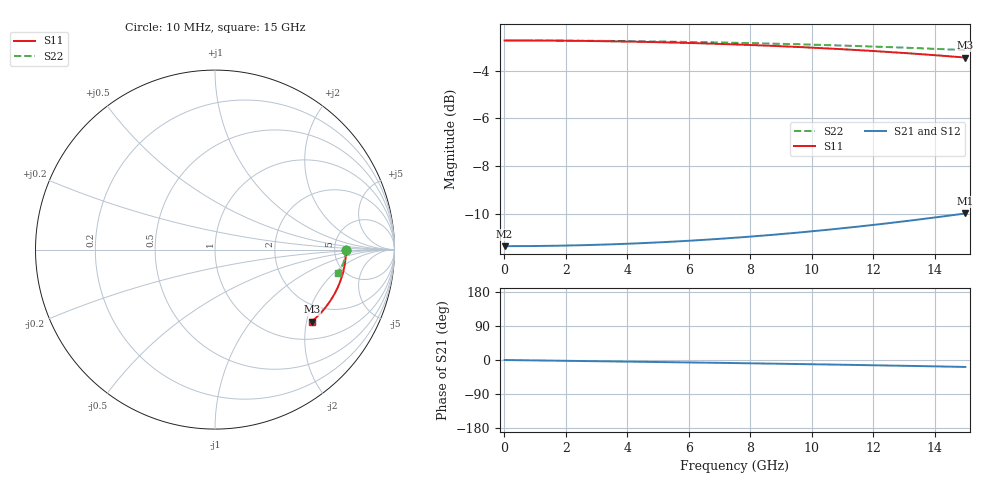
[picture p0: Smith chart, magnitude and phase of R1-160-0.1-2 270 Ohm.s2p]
!version-1
!date-03.2021
# MHz S RI R 50
!Freq ReS11 ImS11 ReS21 ImS21 ReS12 ImS12 ReS22 ImS22
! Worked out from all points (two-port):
!   751 points, 10 MHz to 15 GHz, reference 50 ohm
!   highest |S21| = -9.99 dB at 15 GHz (marker M1); lowest = -11.4 dB at 10 MHz (marker M2)
!   |S21| within 3 dB of the highest: start of sweep to end of sweep
!   lowest |S11| = -3.5 dB at 15 GHz (marker M3), VSWR 5.10, Z = 73.4 - j107 ohm
!   |S11| at or under -10 dB: nowhere
!   |S22| runs from -3.1 to -2.7 dB; largest |S21 - S12| = 0
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10  0.7297 -0.000279  0.2703 -4.85e-05  0.2703 -4.85e-05  0.7297 -8.62e-05
70  0.7297 -0.00195  0.2703 -0.00034  0.2703 -0.00034  0.7297 -0.000603
1270  0.7285 -0.0354  0.2705 -0.00618  0.2705 -0.00618  0.7294 -0.0109
2510  0.7248 -0.07  0.2712 -0.0123  0.2712 -0.0123  0.7285 -0.0216
3770  0.7187 -0.1051  0.2724 -0.0187  0.2724 -0.0187  0.727 -0.0325
5010  0.7101 -0.1395  0.2741 -0.0252  0.2741 -0.0252  0.7248 -0.0431
5650  0.7047 -0.1572  0.2751 -0.0288  0.2751 -0.0288  0.7235 -0.0486
6270  0.6988 -0.1742  0.2762 -0.0323  0.2762 -0.0323  0.7221 -0.0539
6890  0.6922 -0.1913  0.2774 -0.0359  0.2774 -0.0359  0.7205 -0.0593
7510  0.685 -0.2082  0.2787 -0.0396  0.2787 -0.0396  0.7187 -0.0646
8150  0.6768 -0.2256  0.2801 -0.0436  0.2801 -0.0436  0.7167 -0.07
8770  0.6681 -0.2424  0.2816 -0.0476  0.2816 -0.0476  0.7146 -0.0753
9390  0.6588 -0.2591  0.2832 -0.0518  0.2832 -0.0518  0.7124 -0.0806
10010  0.6487 -0.2756  0.2849 -0.0562  0.2849 -0.0562  0.71 -0.0859
10650  0.6375 -0.2926  0.2867 -0.0609  0.2867 -0.0609  0.7073 -0.0913
11270  0.6259 -0.3088  0.2885 -0.0657  0.2885 -0.0657  0.7046 -0.0966
11890  0.6135 -0.3248  0.2904 -0.0706  0.2904 -0.0706  0.7017 -0.1019
12510  0.6003 -0.3406  0.2924 -0.0759  0.2924 -0.0759  0.6986 -0.1071
13110  0.5867 -0.3557  0.2943 -0.0812  0.2943 -0.0812  0.6955 -0.1122
13690  0.5729 -0.37  0.2962 -0.0866  0.2962 -0.0866  0.6923 -0.117
14610  0.5494 -0.3922  0.2992 -0.0956  0.2992 -0.0956  0.687 -0.1248
15000  0.5388 -0.4014  0.3004 -0.0996  0.3004 -0.0996  0.6846 -0.128
